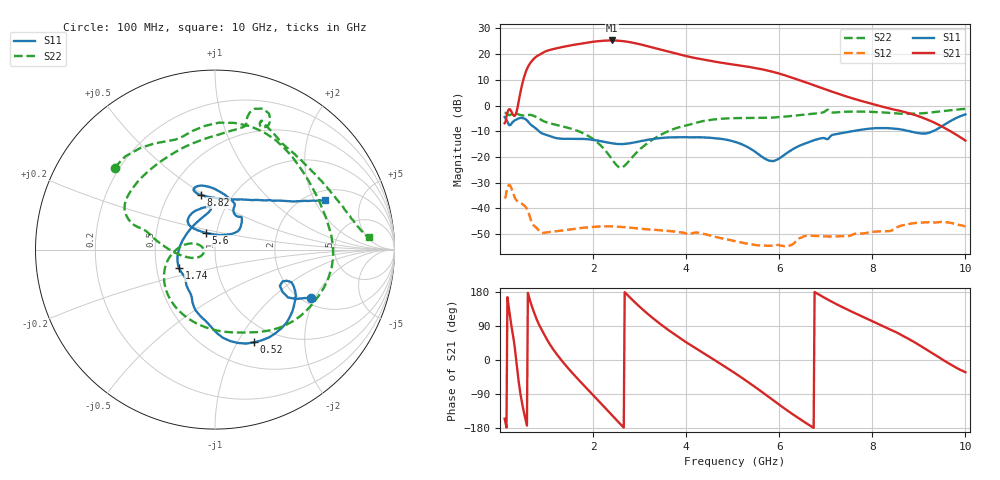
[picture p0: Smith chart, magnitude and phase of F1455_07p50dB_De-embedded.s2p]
! Integrated Device Technology
! Corporate Headquarters
! 6024 Silver Creek Valley Road
! San Jose, CA 95138  USA
! Phone:  1-408-284-8200
! Toll Free:  1-800-223-1366
! Webpage:  http://www.idt.com/
! Timing and RF Division
! 515 Groton Road, Suite 102
! Westford, MA 01886-6024
! Device:  F1455
! Description: 6-bit 0.5 dB Transmit Variable Gain Amplifier
! Frequency:  1400.0 -  2300.00 MHz
! Package:  6x6 mm Thin QFN Plastic Package: 28 pin
! State:  15
! Atten State:  7.5 dB
! Voltage:  +5.00 Volts
! Current:  217.651 mA
! Data:  The device was measured on a the F1455 evaluation board which has
!  individual transmission lines to the RF pins.  Data was collected
!  using a calibrated network analyzer.  The evaluation board was
!  de-embedded using a TRL calibration technique.
!  The reference plane is the edge of the package pin.
!  Pin  1 = CSb
!  Pin  2 = DATA
!  Pin  3 = CLK
!  Pin  4 = RSET
!  Pin  5 = GND
!  Pin  6 = RFIN  = Port 1
!  Pin  7 = GND
!  Pin  8 = NC
!  Pin  9 = NC
!  Pin 10 = NC
!  Pin 11 = NC
!  Pin 12 = NC
!  Pin 13 = NC
!  Pin 14 = /STBY
!  Pin 15 = GND
!  Pin 16 = RFOUT  = Port 2
!  Pin 17 = GND
!  Pin 18 = NC
!  Pin 19 = NC
!  Pin 20 = NC
!  Pin 21 = GND
!  Pin 22 = NC
!  Pin 23 = GND
!  Pin 24 = NC
!  Pin 25 = NC
!  Pin 26 = NC
!  Pin 27 = GND
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# GHz S dB R 50
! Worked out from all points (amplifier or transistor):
!   496 points, 100 MHz to 10 GHz, reference 50 ohm
!   highest |S21| = 25.3 dB at 2.4 GHz (marker M1)
!   |S21| within 3 dB of that: 1.228 GHz to 3.334 GHz (2.106 GHz wide, 92.3 % of centre)
!   unconditionally stable (mu >= 1): start of sweep to end of sweep
!   at 1.74 GHz: K = 6.48, MAG = 24.8 dB, |S12| = -47.6 dB
!   at 5.06 GHz: K = 22.70, MAG = 17.7 dB, |S12| = -52.7 dB
!   at 10 GHz: K = 74.12, MAG = -5.1 dB, |S12| = -46.9 dB
!   S11 on the Smith chart (normalised r, x): 100 MHz: 2.21, -1.86; 520 MHz: 0.78, -1.18; 1.74 GHz: 0.65, -0.14; 5.6 GHz: 0.89, +0.17; 8.82 GHz: 0.72, +0.49; 10 GHz: 2.40, +2.45
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0.1  -4.47 -26.8  -6.85 -155.1  -36.08 43.4  -2.83 140.8
0.38  -5.17 -38.6  -0.52 -34.1  -37.20 -110.0  -3.28 56.1
0.52  -5.02 -67.1  11.16 -141.1  -38.83 -155.6  -3.88 24.2
0.7  -7.96 -97.6  17.62 136.5  -45.99 149.7  -3.83 -19.2
0.82  -9.71 -112.0  19.48 98.5  -48.27 134.0  -4.80 -47.1
0.96  -11.21 -120.8  20.89 65.3  -49.44 123.3  -6.25 -71.6
1.14  -12.31 -132.4  21.94 28.8  -49.02 101.2  -7.21 -96.9
1.34  -12.89 -139.2  22.76 -3.5  -48.56 79.3  -8.07 -120.8
1.74  -12.93 -153.2  24.09 -58.8  -47.62 45.2  -10.36 -158.0
1.76  -12.94 -154.1  24.14 -61.4  -47.57 43.7  -10.52 -159.6
2.08  -13.55 -171.4  24.97 -102.8  -47.09 21.2  -14.13 175.9
2.4  -14.65 160.5  25.31 -144.7  -46.96 0.7  -20.68 163.3
2.66  -14.91 132.2  25.01 -178.5  -47.24 -14.3  -23.65 -164.8
2.94  -14.15 108.1  24.10 147.5  -47.70 -28.0  -18.23 -157.8
3.4  -12.73 95.6  22.00 99.3  -48.45 -46.6  -11.94 -180.0
4.1  -12.34 111.8  18.82 39.1  -49.82 -69.1  -7.30 163.9
5.06  -14.15 136.4  15.83 -35.5  -52.74 -106.0  -4.88 148.8
5.6  -19.55 118.1  14.19 -81.7  -54.38 -113.3  -4.82 127.4
6.7  -13.80 44.1  8.19 -176.1  -50.58 -143.6  -3.22 78.5
8.36  -8.79 108.0  -1.12 81.8  -48.82 162.3  -2.84 62.5
8.82  -10.03 104.5  -3.15 52.8  -45.90 146.6  -3.21 45.1
10  -3.43 24.5  -13.59 -32.2  -46.89 75.7  -1.30 4.7
